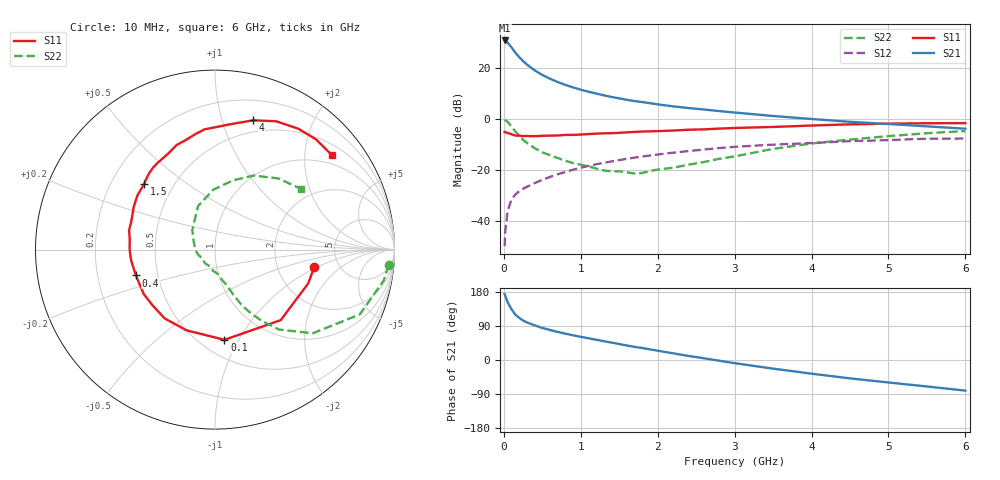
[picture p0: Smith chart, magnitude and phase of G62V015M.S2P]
! SIEMENS Small Signal Semiconductors
! BFG193
! Si NPN RF Bipolar Junction Transistor in SOT223
! VCE = 2 V  IC = 15 mA
! Common Emitter S-Parameters:  August  1996
# GHz  S  MA  R  50
!  f  S11  S21  S12  S22
! GHz  MAG  ANG  MAG  ANG  MAG  ANG  MAG  ANG
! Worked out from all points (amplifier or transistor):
!   36 points, 10 MHz to 6 GHz, reference 50 ohm
!   highest |S21| = 30.9 dB at 10 MHz (marker M1)
!   |S21| within 3 dB of that: start of sweep to 106.9 MHz
!   unconditionally stable (mu >= 1): 731.7 MHz to 2.676 GHz
!   at 250 MHz: K = 0.67, MSG = 25.1 dB, |S12| = -27.4 dB
!   at 1.4 GHz: K = 1.06, MAG = 11.2 dB, |S12| = -16.6 dB
!   at 6 GHz: K = 0.92, MSG = 1.9 dB, |S12| = -7.6 dB
!   S11 on the Smith chart (normalised r, x): 10 MHz: 3.27, -0.93; 100 MHz: 0.65, -0.87; 400 MHz: 0.37, -0.14; 1.5 GHz: 0.34, +0.35; 4 GHz: 0.38, +1.27; 6 GHz: 0.74, +2.63
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0.01  0.5612 -10.0  35.27 173.9  0.0032 91.5  0.9708 -5.1
0.02  0.5527 -19.9  34.86 168.7  0.0066 82.7  0.9563 -10.3
0.05  0.5373 -47.0  31.94 152.2  0.016 70.5  0.8839 -24.1
0.1  0.5053 -84.0  25.8 133.6  0.0266 61.5  0.7165 -40.6
0.15  0.477 -109.5  20.31 119.6  0.0332 55.2  0.5707 -51.3
0.2  0.475 -126.3  16.64 111.1  0.0384 53.7  0.4726 -56.9
0.25  0.4663 -138.6  13.86 104.2  0.0428 53.5  0.3941 -61.3
0.3  0.4679 -148.1  11.86 99.1  0.047 53.7  0.3441 -64.2
0.4  0.4639 -161.9  9.154 91.5  0.0554 54.4  0.2701 -68.0
0.5  0.4711 -172.8  7.397 84.6  0.0643 54.7  0.2242 -70.6
0.6  0.4758 180.0  6.239 79.2  0.0736 55.1  0.1957 -73.3
0.7  0.4782 173.2  5.382 74.1  0.0827 55.1  0.173 -77.0
0.9  0.4916 162.0  4.213 65.2  0.1019 53.4  0.1372 -83.4
1.1  0.5102 152.8  3.465 57.3  0.1207 51.2  0.1187 -95.0
1.5  0.5391 137.1  2.571 42.2  0.157 44.6  0.0947 -124.4
2.2  0.5981 115.1  1.789 17.7  0.22 30.6  0.1112 176.2
2.8  0.6533 99.5  1.444 -1.9  0.2713 17.4  0.1668 139.3
3.5  0.7045 82.8  1.156 -22.8  0.3165 0.6  0.261 111.0
4  0.7512 73.5  1.01 -36.1  0.3402 -9.0  0.3339 91.6
4.5  0.7923 64.5  0.889 -48.5  0.3703 -19.1  0.3974 75.7
5.5  0.8331 47.5  0.724 -69.9  0.414 -42.2  0.5303 48.4
6  0.8373 39.1  0.651 -80.8  0.4178 -55.5  0.5865 35.3
